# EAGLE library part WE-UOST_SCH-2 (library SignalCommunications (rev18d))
WE-UOST Universal Offline Standard Transformer Characteristics Input voltage range 85–265 VAC (125–375 VDC) Output power 12–16 W Designed to comply with EN61558-2-16: Reinforced insulation Creepage and clearance distance >6.5 mm Insulation test voltage 4 kVAC For SMD assembly Applications SMPS with power up to 16 W Auxiliary power supplies Usable with all low power AC/DC ICs like LT3798/99, UCC28610, ViPER & Tiny/Link Switch Details see: http://katalog.we-online.de/en/pbs/WE-UOST? Updated by Dan Xu 2014-07-11 2014 (C) Wurth Elektronik
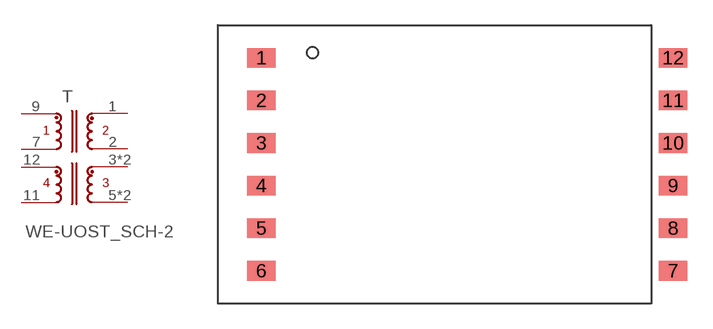
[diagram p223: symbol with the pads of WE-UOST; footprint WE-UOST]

Designator prefix T

## WE-UOST_SCH-2_760871534, WE-UOST_SCH-2_760871543, WE-UOST_SCH-2_760875532  [WE-UOST]
1  1  pas
2  4  pas
3  3  pas
4  3  pas
5  6  pas
6  6  pas
7  7  pas
9  9  pas
11  11  pas
12  12  pas

## Footprint WE-UOST (pad centres in mm)
Universal Offline Standard Transformers WE-UOST
smd 1.7 x 1.17: 1 -12.265,6.35; 2 -12.265,3.81; 3 -12.265,1.27; 4 -12.265,-1.27; 5 -12.265,-3.81; 6 -12.265,-6.35; 7 12.265,-6.35; 8 12.265,-3.81; 9 12.265,-1.27; 10 12.265,1.27; 11 12.265,3.81; 12 12.265,6.35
